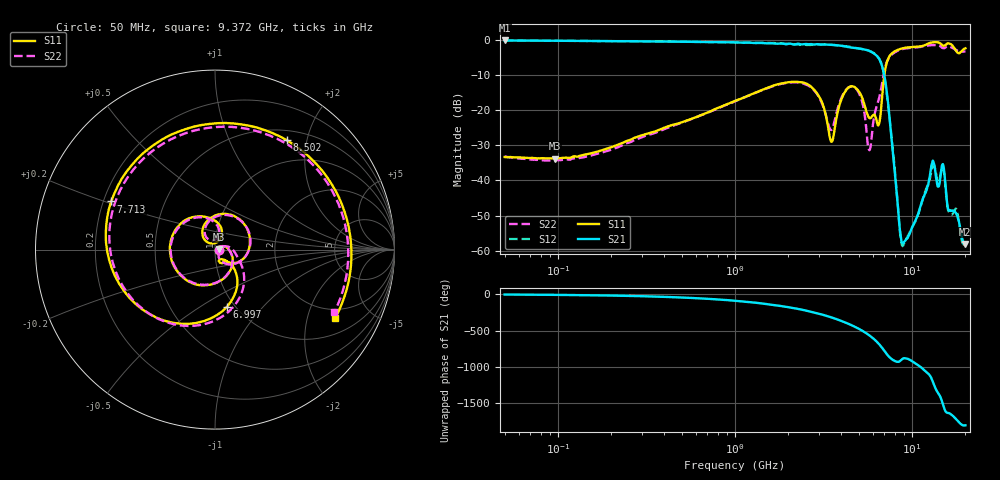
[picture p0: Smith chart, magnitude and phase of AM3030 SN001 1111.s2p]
# Hz S DB R 50
!freq MagS11 AngS11 MagS21 AngS21 MagS12 AngS12 MagS22 AngS22
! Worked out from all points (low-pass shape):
!   1601 points, 50 MHz to 20.05 GHz, reference 50 ohm
!   highest |S21| = -0.27 dB at 50 MHz (marker M1); lowest = -58.1 dB at 19.9 GHz (marker M2)
!   |S21| within 3 dB of the highest: start of sweep to 5.767 GHz
!   lowest |S11| = -33.8 dB at 95.95 MHz (marker M3), VSWR 1.04, Z = 52.1 + j0.311 ohm
!   |S11| at or under -10 dB: start of sweep to 6.987 GHz
!   |S22| runs from -34.4 to -1.5 dB; largest |S21 - S12| = 0.032
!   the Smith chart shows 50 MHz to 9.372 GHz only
!   S11 on the Smith chart (normalised r, x): 50 MHz: 1.04, -0.00; 6.997 GHz: 0.92, -0.66; 7.713 GHz: 0.23, +0.21; 8.502 GHz: 0.64, +1.66; 9.372 GHz: 1.59, -2.99
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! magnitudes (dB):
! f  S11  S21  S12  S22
! 50 MHz  -33.4  -0.3  -0.3  -33.2
! 95.95 MHz  -33.8  -0.4  -0.4  -34.3
! 135.9 MHz  -32.9  -0.4  -0.4  -33.5
! 369.6 MHz  -25.7  -0.6  -0.6  -26.1
! 1.005 GHz  -17.4  -0.8  -0.8  -17.5
! 2.722 GHz  -13.6  -1.3  -1.5  -13.8
! 3.512 GHz  -29.0  -1.5  -1.5  -25.7
! 4.095 GHz  -15.8  -1.9  -1.8  -15.4
! 4.811 GHz  -13.7  -2.4  -2.4  -13.8
! 5.759 GHz  -22.3  -3.3  -3.2  -31.4
! 6.492 GHz  -24.2  -5.3  -5.3  -17.1
! 6.997 GHz  -9.8  -10.5  -10.8  -8.8
! 7.402 GHz  -5.1  -20.0  -20.2  -5.3
! 7.713 GHz  -3.9  -28.9  -28.7  -4.2
! 8.502 GHz  -2.7  -53.0  -53.2  -3.0
! 9.372 GHz  -2.3  -56.6  -56.3  -2.5
! 13.13 GHz  -0.8  -34.4  -36.0  -1.6
! 14.05 GHz  -0.8  -41.8  -40.1  -1.6
! 14.97 GHz  -1.7  -35.4  -36.2  -2.4
! 16.19 GHz  -1.1  -48.5  -49.0  -2.0
! 19.9 GHz  -2.6  -58.1  -58.2  -3.4
! 20.05 GHz  -2.5  -57.9  -58.2  -3.4
